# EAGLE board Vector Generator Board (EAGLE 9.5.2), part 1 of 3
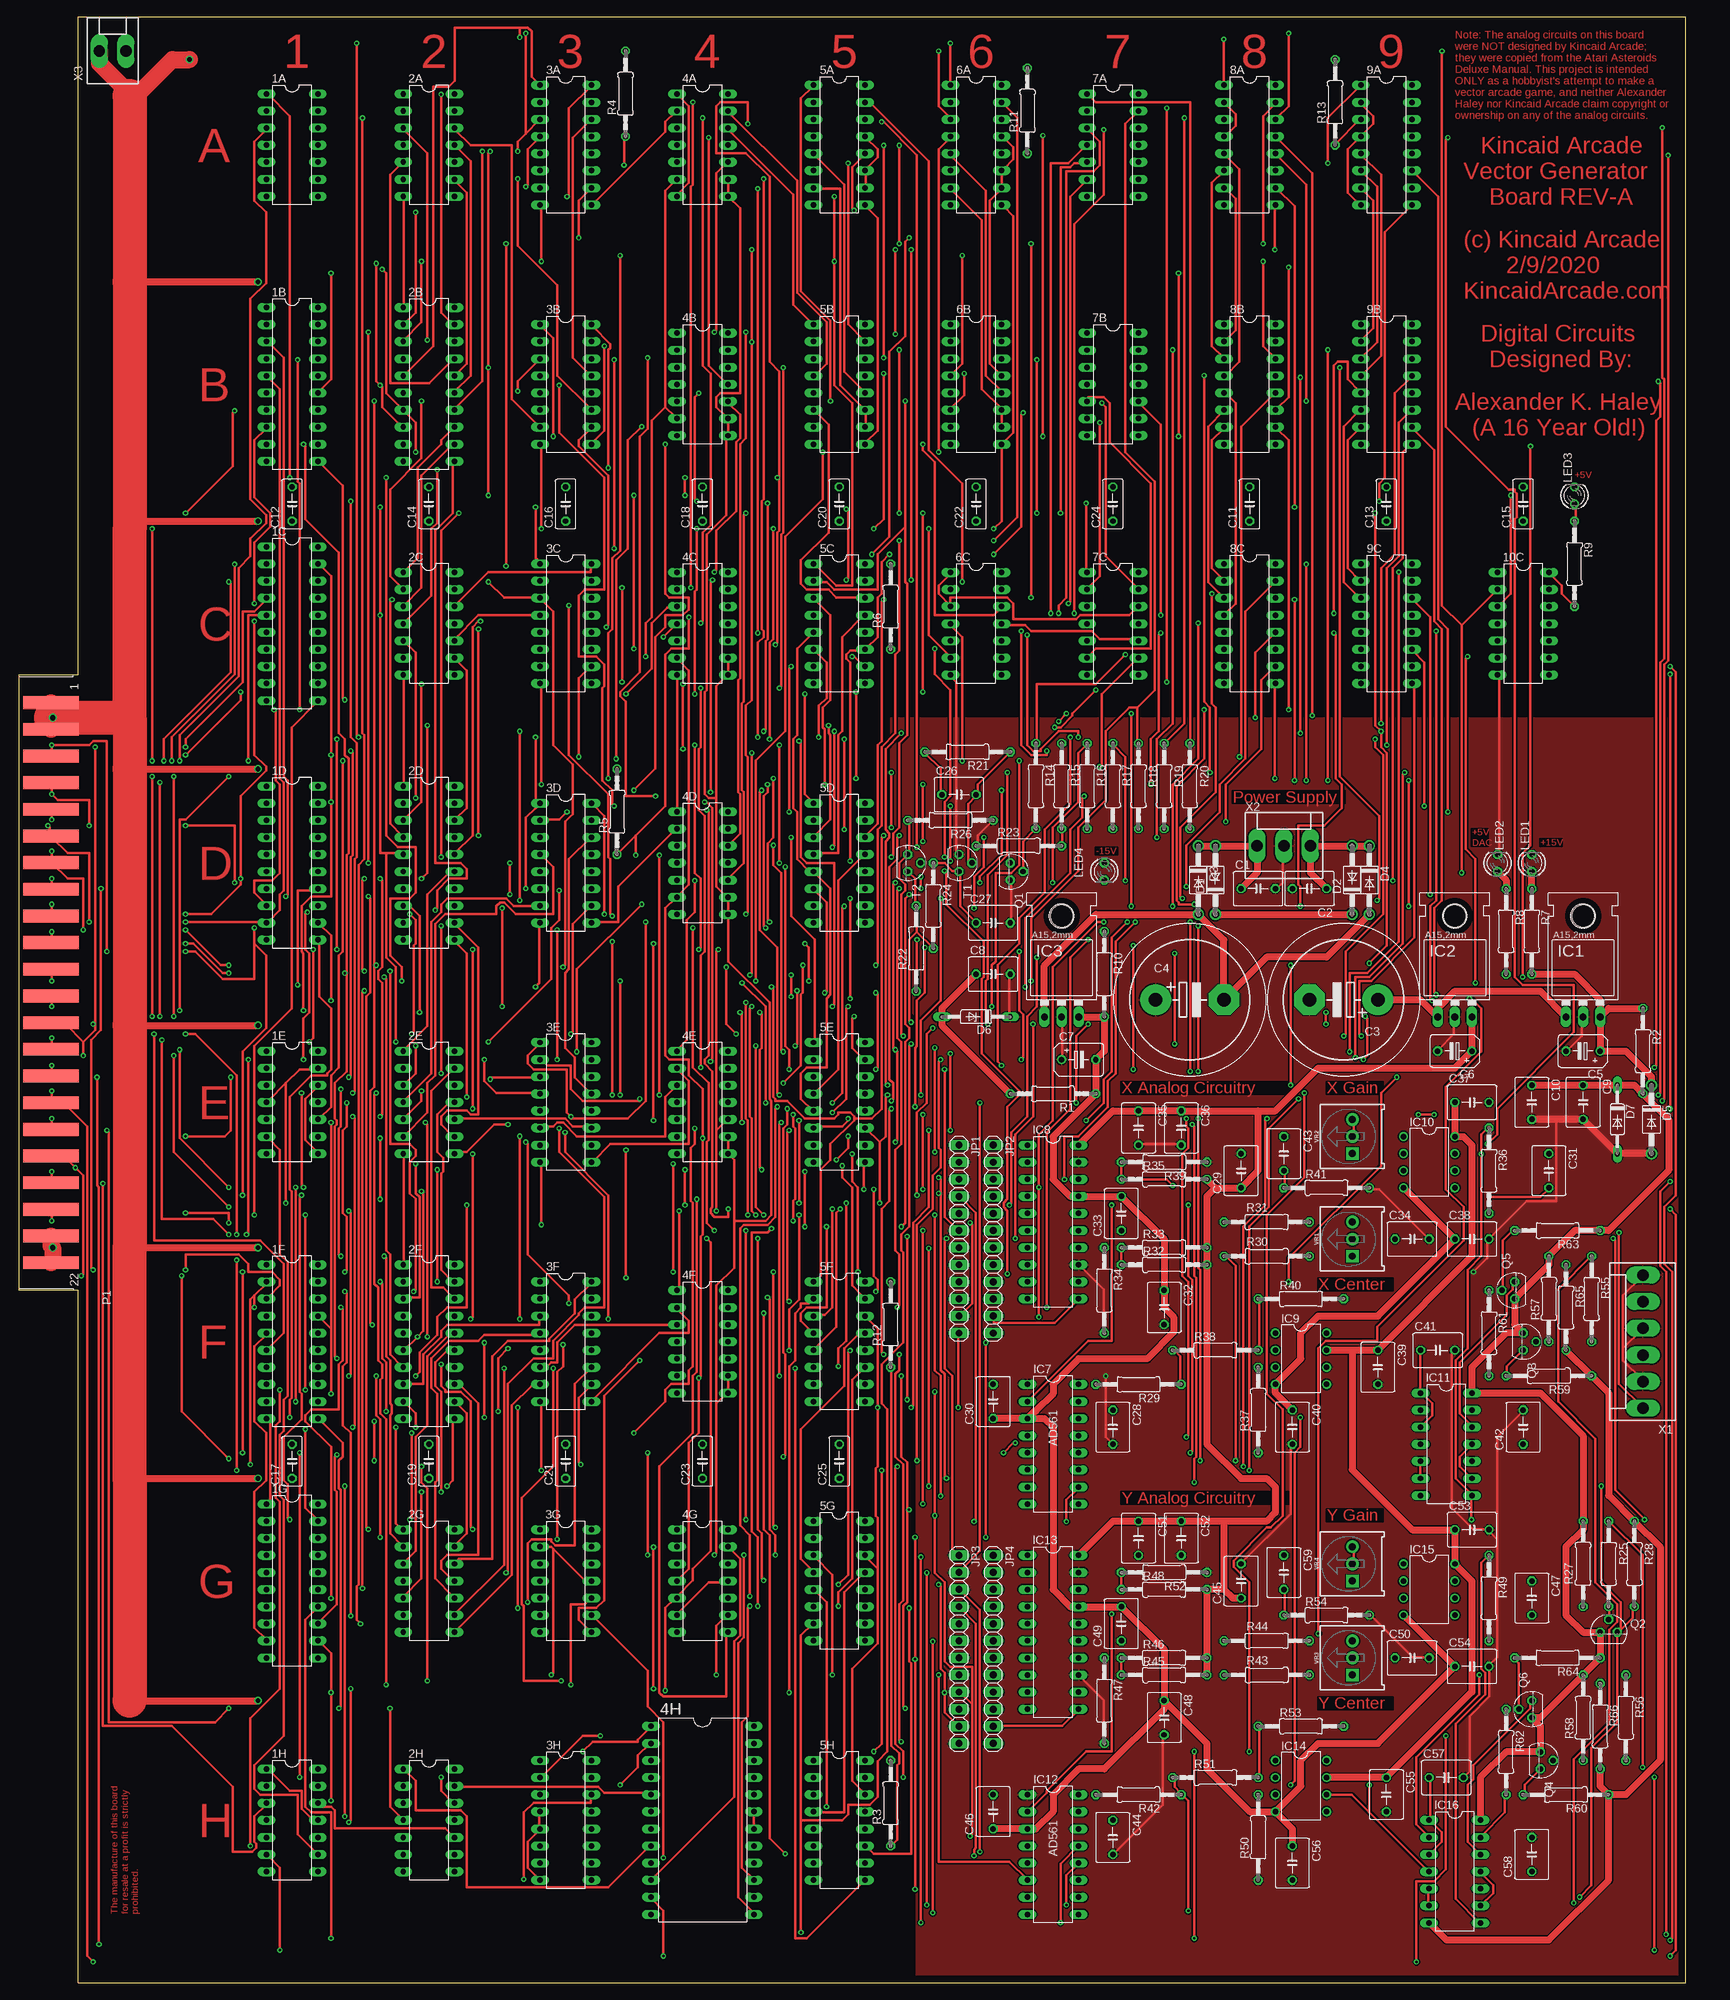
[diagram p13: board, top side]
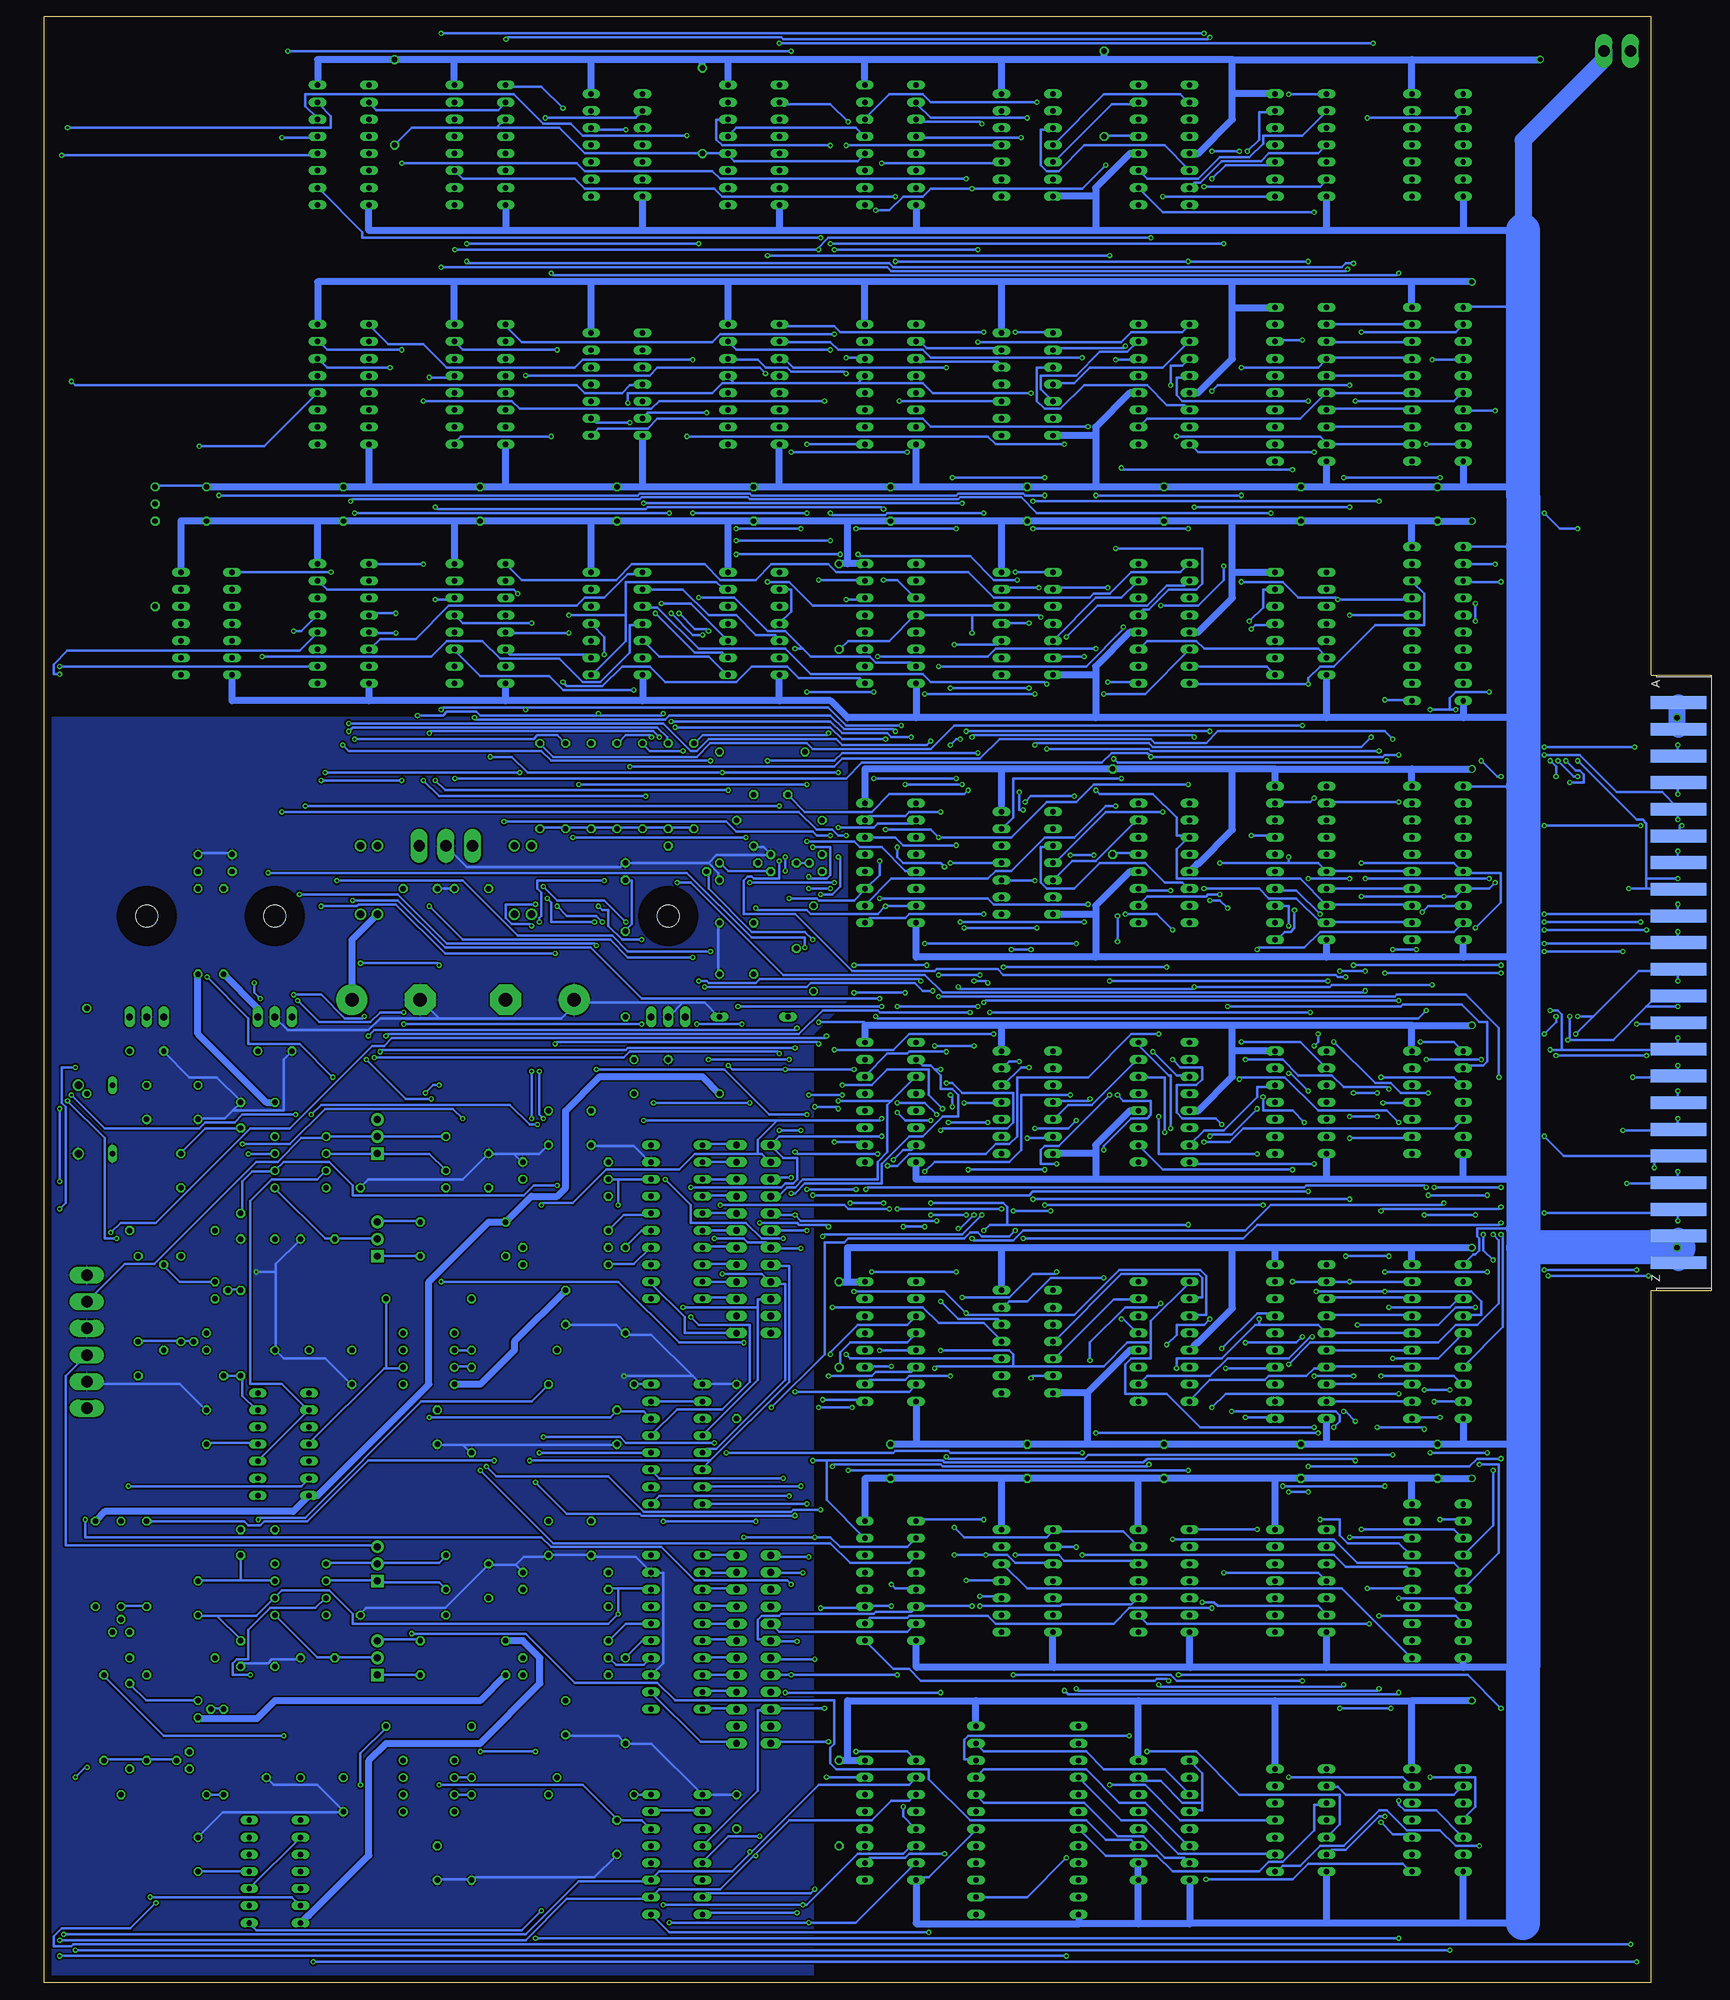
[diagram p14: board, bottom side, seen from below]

Size 247.65 x 292.1 mm. Coordinates in mm from the lower left corner, seen from the top.
Outline: 8.89,0 8.89,102.87 0,102.87 0,194.31 8.89,194.31 8.89,292.1 247.65,292.1 247.65,0 8.89,0
Copper layers (1*16): Top 0.035mm / dielectric 1.5mm / Bottom 0.035mm
Design rules "default": minimum track width 6mil, minimum drill 0.35mm, track to track 6mil, track to pad 6mil, pad to pad 6mil, via to via 6mil, smd to smd 6mil, copper to edge 40mil, drill to drill 6mil, minimum pad ring 10mil, minimum via ring 8mil, stop-mask expansion 4mil, vias tented up to drill 0mil, thermal gap 10mil
Net classes: 0 default: width 0.381 mm, clearance 0.203 mm

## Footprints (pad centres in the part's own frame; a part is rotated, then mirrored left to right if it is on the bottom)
DIL14 = drill 0.813 long: 1 -7.62,-3.81; 2 -5.08,-3.81; 3 -2.54,-3.81; 4 0,-3.81; 5 2.54,-3.81; 6 5.08,-3.81; 7 7.62,-3.81; 8 7.62,3.81; 9 5.08,3.81; 10 2.54,3.81; 11 0,3.81; 12 -2.54,3.81; 13 -5.08,3.81; 14 -7.62,3.81
DIL20 = drill 0.813 long: 1 -11.43,-3.81; 2 -8.89,-3.81; 3 -6.35,-3.81; 4 -3.81,-3.81; 5 -1.27,-3.81; 6 1.27,-3.81; 7 3.81,-3.81; 8 6.35,-3.81; 9 8.89,-3.81; 10 11.43,-3.81; 11 11.43,3.81; 12 8.89,3.81; 13 6.35,3.81; 14 3.81,3.81; 15 1.27,3.81; 16 -1.27,3.81; 17 -3.81,3.81; 18 -6.35,3.81; 19 -8.89,3.81; 20 -11.43,3.81
DIL16 = drill 0.813 long: 1 -8.89,-3.81; 2 -6.35,-3.81; 3 -3.81,-3.81; 4 -1.27,-3.81; 5 1.27,-3.81; 6 3.81,-3.81; 7 6.35,-3.81; 8 8.89,-3.81; 9 8.89,3.81; 10 6.35,3.81; 11 3.81,3.81; 12 1.27,3.81; 13 -1.27,3.81; 14 -3.81,3.81; 15 -6.35,3.81; 16 -8.89,3.81
DIL24-6 = drill 0.813 long: 1 -13.97,-7.62; 2 -11.43,-7.62; 3 -8.89,-7.62; 4 -6.35,-7.62; 5 -3.81,-7.62; 6 -1.27,-7.62; 7 1.27,-7.62; 8 3.81,-7.62; 9 6.35,-7.62; 10 8.89,-7.62; 11 11.43,-7.62; 12 13.97,-7.62; 13 13.97,7.62; 14 11.43,7.62; 15 8.89,7.62; 16 6.35,7.62; 17 3.81,7.62; 18 1.27,7.62; 19 -1.27,7.62; 20 -3.81,7.62; 21 -6.35,7.62; 22 -8.89,7.62; 23 -11.43,7.62; 24 -13.97,7.62
C050-050X075 = drill 0.813 octagon: 1 -2.54,0; 2 2.54,0
EB22,5D = drill 2.007 pad 4.597: + -5.08,0 | drill 2.007 pad 4.597 octagon: - 5.08,0
B45181B = drill 0.813: + -2.54,0 | drill 0.813 octagon: - 2.54,0
C050-030X075 = drill 0.813 octagon: 1 -2.54,0; 2 2.54,0
DO41-10 = drill 1.118: A 5.08,0; C -5.08,0
DO35Z10 = drill 0.813 long: A 5.08,0; C -5.08,0
78XXL = drill 1.016 long: GND 0,-3.81; IN -2.54,-3.81; OUT 2.54,-3.81 | hole 3.302: 0,11.176
DIL08 = drill 0.813 pad 1.27: 1 -3.81,-3.81; 2 -1.27,-3.81; 3 1.27,-3.81; 4 3.81,-3.81; 5 3.81,3.81; 6 1.27,3.81; 7 -1.27,3.81; 8 -3.81,3.81
1X12 = drill 1.016 long: 1 -13.97,0; 2 -11.43,0; 3 -8.89,0; 4 -6.35,0; 5 -3.81,0; 6 -1.27,0; 7 1.27,0; 8 3.81,0; 9 6.35,0; 10 8.89,0; 11 11.43,0; 12 13.97,0
LED3MM = drill 0.813 octagon: A -1.27,0; K 1.27,0
44PINEDGE = smd 1.905 x 8.255: 1 -41.605,4.826; 2 -37.643,4.826; 3 -33.68,4.826; 4 -29.718,4.826; 5 -25.756,4.826; 6 -21.793,4.826; 7 -17.831,4.826; 8 -13.868,4.826; 9 -9.906,4.826; 10 -5.944,4.826; 11 -1.981,4.826; 12 1.981,4.826; 13 5.944,4.826; 14 9.906,4.826; 15 13.868,4.826; 16 17.831,4.826; 17 21.793,4.826; 18 25.756,4.826; 19 29.718,4.826; 20 33.68,4.826; 21 37.643,4.826; 22 41.605,4.826 | smd 1.905 x 8.255 bottom: A -41.605,4.826; B -37.643,4.826; C -33.68,4.826; D -29.718,4.826; E -25.756,4.826; F -21.793,4.826; H -17.831,4.826; J -13.868,4.826; K -9.906,4.826; L -5.944,4.826; M -1.981,4.826; N 1.981,4.826; P 5.944,4.826; R 9.906,4.826; S 13.868,4.826; T 17.831,4.826; U 21.793,4.826; V 25.756,4.826; W 29.718,4.826; X 33.68,4.826; Y 37.643,4.826; Z 41.605,4.826
TO92 = drill 0.813 octagon: 1 1.27,0; 2 0,1.905; 3 -1.27,0
0207/12 = drill 0.813 octagon: 1 -6.35,0; 2 6.35,0
TRIMPOT-PTH-3386U = drill 1.016 pad 1.88 square: 1 -2.54,-0.015 | drill 1.016 pad 1.88: 2 0,-0.015; 3 2.54,-0.015
KK-156-6 = drill 1.7 pad 2.184 long: 1 -9.9,0; 2 -5.94,0; 3 -1.98,0; 4 1.98,0; 5 5.94,0; 6 9.9,0
KK-156-3 = drill 1.7 pad 2.184 long: 1 -3.96,0; 2 0,0; 3 3.96,0
KK-156-2 = drill 1.7 pad 2.184 long: 1 -1.98,0; 2 1.98,0

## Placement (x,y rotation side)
1A  7400N  [DIL14]  40.64,273.05 270 top
1B  74HC573N  [DIL20]  40.64,237.49 270 top
1C  74HC573N  [DIL20]  40.64,201.93 270 top
1D  74HC573N  [DIL20]  40.64,166.37 270 top
1E  74S08N  [DIL14]  40.64,130.81 270 top
1F  74HC573N  [DIL20]  40.64,95.25 270 top
1G  74HC573N  [DIL20]  40.64,59.69 270 top
1H  7432N  [DIL14]  40.64,24.13 270 top
2A  7404N  [DIL14]  60.96,273.05 270 top
2B  74HC573N  [DIL20]  60.96,237.49 270 top
2C  7404N  [DIL14]  60.96,201.93 270 top
2D  74HC573N  [DIL20]  60.96,166.37 270 top
2E  7404N  [DIL14]  60.96,130.81 270 top
2F  74HC573N  [DIL20]  60.96,95.25 270 top
2G  7404N  [DIL14]  60.96,59.69 270 top
2H  7404N  [DIL14]  60.96,24.13 270 top
3A  7483N  [DIL16]  81.28,273.05 270 top
3B  7483N  [DIL16]  81.28,237.49 270 top
3C  7483N  [DIL16]  81.28,201.93 270 top
3D  7483N  [DIL16]  81.28,166.37 270 top
3E  7483N  [DIL16]  81.28,130.81 270 top
3F  7483N  [DIL16]  81.28,95.25 270 top
3G  74S11N  [DIL14]  81.28,59.69 270 top
3H  74191N  [DIL16]  81.28,24.13 270 top
4A  7495N  [DIL14]  101.6,273.05 270 top
4B  7495N  [DIL14]  101.6,237.49 270 top
4C  7495N  [DIL14]  101.6,201.93 270 top
4D  7495N  [DIL14]  101.6,166.37 270 top
4E  7495N  [DIL14]  101.6,130.81 270 top
4F  7495N  [DIL14]  101.6,95.25 270 top
4G  7404N  [DIL14]  101.6,59.69 270 top
4H  74154N  [DIL24-6]  101.6,24.13 270 top
5A  7497N  [DIL16]  121.92,273.05 270 top
5B  7497N  [DIL16]  121.92,237.49 270 top
5C  74191N  [DIL16]  121.92,201.93 270 top
5D  74191N  [DIL16]  121.92,166.37 270 top
5E  74191N  [DIL16]  121.92,130.81 270 top
5F  74191N  [DIL16]  121.92,95.25 270 top
5G  74191N  [DIL16]  121.92,59.69 270 top
5H  74191N  [DIL16]  121.92,24.13 270 top
6A  7497N  [DIL16]  142.24,273.05 270 top
6B  7497N  [DIL16]  142.24,237.49 270 top
6C  74S11N  [DIL14]  142.24,201.93 270 top
7A  74LS27N  [DIL14]  162.56,273.05 270 top
7B  7432N  [DIL14]  162.56,237.49 270 top
7C  7404N  [DIL14]  162.56,201.93 270 top
8A  7485N  [DIL16]  182.88,273.05 270 top
8B  7485N  [DIL16]  182.88,237.49 270 top
8C  7485N  [DIL16]  182.88,201.93 270 top
9A  7485N  [DIL16]  203.2,273.05 270 top
9B  7485N  [DIL16]  203.2,237.49 270 top
9C  7485N  [DIL16]  203.2,201.93 270 top
10C  7402N  [DIL14]  223.52,201.93 270 top
C1  .1 uf  [C050-050X075]  184.15,162.56 0 top
C2  .1 uf  [C050-050X075]  191.77,162.56 180 top
C3  470 uf  [EB22,5D]  196.85,146.05 180 top
C4  470 uf  [EB22,5D]  173.99,146.05 0 top
C5  1 uf  [B45181B]  232.41,138.43 180 top
C6  1 uf  [B45181B]  213.36,138.43 180 top
C7  1 uf  [B45181B]  157.48,137.16 0 top
C8  .1 uf  [C050-050X075]  144.78,149.86 0 top
C9  .1 uf  [C050-050X075]  232.41,130.81 270 top
C10  22pf  [C050-050X075]  224.79,130.81 270 top
C11  .1uf  [C050-030X075]  182.88,219.71 90 top
C12  .1uf  [C050-030X075]  40.64,219.71 90 top
C13  .1uf  [C050-030X075]  203.2,219.71 90 top
C14  .1uf  [C050-030X075]  60.96,219.71 90 top
C15  .1uf  [C050-030X075]  223.52,219.71 90 top
C16  .1uf  [C050-030X075]  81.28,219.71 90 top
C17  .1uf  [C050-030X075]  40.64,77.47 90 top
C18  .1uf  [C050-030X075]  101.6,219.71 90 top
C19  .1uf  [C050-030X075]  60.96,77.47 90 top
C20  .1uf  [C050-030X075]  121.92,219.71 90 top
C21  .1uf  [C050-030X075]  81.28,77.47 90 top
C22  .1uf  [C050-030X075]  142.24,219.71 90 top
C23  .1uf  [C050-030X075]  101.6,77.47 90 top
C24  .1uf  [C050-030X075]  162.56,219.71 90 top
C25  .1uf  [C050-030X075]  121.92,77.47 90 top
C26  270pf  [C050-050X075]  139.7,176.53 0 top
C27  .01uf  [C050-050X075]  144.78,157.48 0 top
C28  .1uf  [C050-050X075]  162.56,82.55 270 top
C29  .1uf  [C050-050X075]  181.61,120.65 90 top
C30  .1uf  [C050-050X075]  144.78,86.36 90 top
C31  10pf  [C050-050X075]  227.33,120.65 270 top
C32  .1uf  [C050-050X075]  170.18,100.33 270 top
C33  .01uf  [C050-050X075]  163.83,114.3 90 top
C34  .1uf  [C050-050X075]  207.01,110.49 0 top
C35  .1uf  [C050-050X075]  166.37,127 270 top
C36  .1uf  [C050-050X075]  172.72,127 270 top
C37  .1uf  [C050-050X075]  215.9,130.81 0 top
C38  .1uf  [C050-050X075]  215.9,110.49 0 top
C39  .1uf  [C050-050X075]  201.93,91.44 270 top
C40  .1uf  [C050-050X075]  189.23,82.55 270 top
C41  220pf  [C050-050X075]  210.82,93.98 0 top
C42  220pf  [C050-050X075]  223.52,82.55 90 top
C43  69pf  [C050-050X075]  187.96,123.19 270 top
C44  .1uf  [C050-050X075]  162.56,21.59 270 top
C45  .1uf  [C050-050X075]  181.61,59.69 90 top
C46  .1uf  [C050-050X075]  144.78,25.4 90 top
C47  10pf  [C050-050X075]  224.79,57.15 270 top
C48  .1uf  [C050-050X075]  170.18,39.37 270 top
C49  .01uf  [C050-050X075]  163.83,53.34 90 top
C50  .1uf  [C050-050X075]  207.01,48.26 0 top
C51  .1uf  [C050-050X075]  166.37,66.04 270 top
C52  .1uf  [C050-050X075]  172.72,66.04 270 top
C53  .1uf  [C050-050X075]  215.9,67.31 0 top
C54  .1uf  [C050-050X075]  215.9,46.99 0 top
C55  .1uf  [C050-050X075]  203.2,27.94 270 top
C56  .1uf  [C050-050X075]  189.23,17.78 270 top
C57  220pf  [C050-050X075]  212.09,30.48 0 top
C58  220pf  [C050-050X075]  224.79,19.05 90 top
C59  69pf  [C050-050X075]  187.96,60.96 270 top
D1  1N4004  [DO41-10]  177.8,163.83 90 top
D2  1N4004  [DO41-10]  198.12,163.83 90 top
D3  1N4004  [DO41-10]  175.26,163.83 270 top
D4  1N4004  [DO41-10]  200.66,163.83 270 top
D5  NTE109  [DO41-10]  242.57,128.27 270 top
D6  NTE5016  [DO35Z10]  142.24,143.51 180 top
D7  1n756a  [DO35Z10]  237.49,128.27 270 top
IC1  7815  [78XXL]  232.41,147.32 0 top
IC2  7805  [78XXL]  213.36,147.32 0 top
IC3  7915  [78XXL]  154.94,147.32 0 top
IC7  AD561  [DIL16]  153.67,80.01 270 top
IC8  DAC312  [DIL20]  153.67,113.03 270 top
IC9  TL081P  [DIL08]  190.5,92.71 270 top
IC10  TL082P  [DIL08]  209.55,121.92 270 top
IC11  4016N  [DIL14]  212.09,80.01 270 top
IC12  AD561  [DIL16]  153.67,19.05 270 top
IC13  DAC312  [DIL20]  153.67,52.07 270 top
IC14  TL081P  [DIL08]  190.5,29.21 270 top
IC15  TL082P  [DIL08]  209.55,58.42 270 top
IC16  4016N  [DIL14]  213.36,16.51 270 top
JP1  [1X12]  139.7,110.49 270 top
JP2  [1X12]  144.78,110.49 270 top
JP3  [1X12]  139.7,49.53 270 top
JP4  [1X12]  144.78,49.53 270 top
LED1  [LED3MM]  224.79,166.37 90 top
LED2  [LED3MM]  219.71,166.37 90 top
LED3  [LED3MM]  231.14,220.98 90 top
LED4  [LED3MM]  161.29,165.1 270 top
P1  44PINEDGE  [44PINEDGE]  0,148.59 270 top
Q1  2N3906  [TO92]  147.32,165.1 270 top
Q2  2N3906  [TO92]  236.22,52.07 0 top
Q3  2N3906  [TO92]  223.52,95.25 270 top
Q4  2N3906  [TO92]  226.06,33.02 270 top
Q5  2N3906  [TO92]  222.25,102.87 90 top
Q6  2N3906  [TO92]  224.79,40.64 90 top
R1  270  [0207/12]  153.67,132.08 180 top
R2  270  [0207/12]  241.3,138.43 270 top
R3  1K  [0207/12]  129.54,26.67 90 top
R4  1K  [0207/12]  90.17,280.67 90 top
R5  1K  [0207/12]  88.9,173.99 90 top
R6  1K  [0207/12]  129.54,204.47 90 top
R7  680  [0207/12]  224.79,156.21 270 top
R8  150  [0207/12]  220.98,156.21 270 top
R9  150  [0207/12]  231.14,210.82 270 top
R10  680  [0207/12]  161.29,149.86 270 top
R11  1K  [0207/12]  149.86,278.13 90 top
R12  1K  [0207/12]  129.54,97.79 90 top
R13  1K  [0207/12]  195.58,279.4 90 top
R14  1.2K  [0207/12]  151.13,177.8 270 top
R15  2.2K  [0207/12]  154.94,177.8 270 top
R16  4.7K  [0207/12]  158.75,177.8 270 top
R17  10K  [0207/12]  162.56,177.8 270 top
R18  22K  [0207/12]  166.37,177.8 270 top
R19  47K  [0207/12]  170.18,177.8 270 top
R20  82K  [0207/12]  173.99,177.8 270 top
R21  1K  [0207/12]  140.97,182.88 180 top
R22  12K  [0207/12]  133.35,153.67 90 top
R23  150K  [0207/12]  148.59,168.91 0 top
R24  68  [0207/12]  135.89,160.02 270 top
R25  18K  [0207/12]  236.22,62.23 270 top
R26  27  [0207/12]  138.43,172.72 180 top
R27  2.2K  [0207/12]  232.41,62.23 90 top
R28  3.3K  [0207/12]  240.03,62.23 270 top
R29  2.2K  [0207/12]  166.37,88.9 180 top
R30  56K  [0207/12]  185.42,107.95 180 top
R31  56K  [0207/12]  185.42,113.03 0 top
R32  10k  [0207/12]  170.18,106.68 0 top
R33  10k  [0207/12]  170.18,109.22 0 top
R34  4.7K  [0207/12]  161.29,102.87 270 top
R35  10K  [0207/12]  170.18,119.38 0 top
R36  8.2K  [0207/12]  218.44,120.65 270 top
R37  4.7K  [0207/12]  184.15,85.09 90 top
R38  10K  [0207/12]  177.8,93.98 0 top
R39  2.2K  [0207/12]  170.18,121.92 180 top
R40  10K  [0207/12]  190.5,101.6 0 top
R41  3.9K  [0207/12]  194.31,118.11 0 top
R42  2.2K  [0207/12]  166.37,27.94 180 top
R43  56K  [0207/12]  185.42,45.72 180 top
R44  56K  [0207/12]  185.42,50.8 0 top
R45  10k  [0207/12]  170.18,45.72 0 top
R46  10k  [0207/12]  170.18,48.26 0 top
R47  4.7K  [0207/12]  161.29,41.91 270 top
R48  10K  [0207/12]  170.18,58.42 0 top
R49  8.2K  [0207/12]  218.44,57.15 270 top
R50  4.7K  [0207/12]  184.15,21.59 90 top
R51  10K  [0207/12]  177.8,30.48 0 top
R52  2.2K  [0207/12]  170.18,60.96 180 top
R53  10K  [0207/12]  190.5,38.1 0 top
R54  3.9K  [0207/12]  194.31,54.61 0 top
R55  18K  [0207/12]  233.68,101.6 270 top
R56  18K  [0207/12]  238.76,39.37 270 top
R57  2.2K  [0207/12]  227.33,101.6 90 top
R58  2.2K  [0207/12]  232.41,39.37 90 top
R59  3.3K  [0207/12]  227.33,90.17 180 top
R60  3.3K  [0207/12]  229.87,27.94 180 top
R61  100K  [0207/12]  218.44,96.52 270 top
R62  100K  [0207/12]  220.98,34.29 270 top
R63  4.7K  [0207/12]  228.6,111.76 180 top
R64  4.7K  [0207/12]  228.6,48.26 180 top
R65  56K  [0207/12]  229.87,100.33 270 top
R66  56K  [0207/12]  234.95,38.1 270 top
T1  2N3904  [TO92]  139.7,166.37 270 top
T2  2N3904  [TO92]  132.08,166.37 270 top
VR1  10k  [TRIMPOT-PTH-3386U]  198.12,110.49 90 top
VR2  10k  [TRIMPOT-PTH-3386U]  198.12,125.73 90 top
VR3  10k  [TRIMPOT-PTH-3386U]  198.12,48.26 90 top
VR4  10k  [TRIMPOT-PTH-3386U]  198.12,62.23 90 top
X1  [KK-156-6]  241.3,95.25 90 top
X2  [KK-156-3]  187.96,168.91 0 top
X3  [KK-156-2]  13.97,287.02 0 top

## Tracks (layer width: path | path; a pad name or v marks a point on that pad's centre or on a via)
2.5MHZ  (via drill 0.35)
  Top 0.381: v103.67,45.73 103.67,53.04 105.13,54.5 4G.9 | v60.73,44.86 60.73,73.48 59.86,74.36 v59.86,76.69 | v31.23,77.86 24.22,84.87 v24.22,105.03 | v9.32,105.03 9.61,105.32 9.61,119.93 v8.45,121.09 6.98,122.56 4.94,122.56 P1.18 | v140.18,181.56 140.18,199.96 138.43,201.71 6C.4 | v108.93,182.73 108.93,150.01 v108.64,149.72 | v114.77,146.51 v114.77,149.72 | v31.52,134.53 31.52,126.64 30.64,125.77 v24.8,125.77
  Bottom 0.381: v103.67,45.73 80.3,45.73 79.43,44.86 v60.73,44.86 | v59.86,76.69 35.9,76.69 34.73,77.86 v31.23,77.86 | v9.32,105.03 v24.22,105.03 | 6C.4 138.43,202.01 136.68,203.76 136.68,206.97 138.43,206.97 6C.2 | v140.18,181.56 130.25,181.56 129.08,182.73 v108.93,182.73 | v114.77,149.72 v108.64,149.72 | v114.77,146.51 47,146.51 46.71,146.8 36.49,146.8 31.52,141.83 v31.52,134.53 | v24.8,125.77 21.88,122.85 8.45,122.85 | 8.45,122.85 4.94,122.85 P1.18 8.45,122.85 | 8.45,122.85 v8.45,121.09
20MHZ  (via drill 0.35)
  Top 0.381: 79.43,64.43 84.1,59.75 84.98,59.75 3G.11 | 79.43,64.43 79.13,64.72 77.67,64.72 3G.2 | 79.43,64.43 79.43,46.02 v79.13,45.73 | v31.23,40.77 29.18,38.72 13.41,38.72 13.41,126.35 v13.12,126.64 | v4.94,128.4 4.94,126.94 P1.17
  Bottom 0.381: v79.13,45.73 36.2,45.73 v31.23,40.77 | v13.12,126.64 4.94,126.64 P1.17 4.94,126.94 v4.94,128.4
25VAC_A
  Top 1.016: D3.C D1.A X2.1 184,164.95 C1.1
25VAC_B
  Top 1.016: C2.1 191.92,164.95 X2.3 D2.A D4.C
+5V_DAC
  Top 1.016: IC2.OUT C6.+ 213.36,135.89 193.04,135.89 186.69,129.54 184.15,129.54 | 184.15,129.54 184.15,120.65 C29.1 177.8,118.11 | 184.15,129.54 C36.1 C35.1 162.56,129.54 IC8.20 | R35.2 177.8,118.11 | 177.8,118.11 176.53,116.84 R33.2 R32.2 176.53,80.01 181.61,74.93 185.42,74.93 186.69,73.66 186.69,69.85 185.42,68.58 179.07,68.58 | 179.07,68.58 C52.1 C51.1 162.56,68.58 IC13.20 | 179.07,68.58 179.07,58.42 | 179.07,58.42 R48.2 R46.2 R45.2 | 179.07,58.42 180.34,57.15 C45.1
  Bottom 1.016: IC2.OUT 215.9,144.78 R8.2
+5VDC  (via drill 0.35)
  Top 0.381: v188.96,29.38 189.55,29.96 189.55,78.74 190.42,79.62 v190.42,84
  Bottom 0.381: IC12.14 157.71,22.95 158.88,24.12 162.38,24.12 C44.1 162.67,24.41 167.64,29.38 v188.96,29.38 | IC7.14 157.71,84 158.59,84.87 162.38,84.87 C28.1 162.67,84.87 163.55,84 v190.42,84
+8.2VDC  (via drill 0.35)
  Top 0.381: v180.78,77.57 180.78,106.49 179.32,107.95 R30.2
  Top 1.016: C10.1 C9.1 D7.C 240.03,133.35 R2.2 245.11,128.27 245.11,120.65 236.22,111.76 R63.1 231.14,111.76 R57.2 227.33,106.68 Q5.3 222.25,97.79 Q3.3 220.98,96.52 215.9,91.44 IC11.14 226.06,87.63 232.41,81.28 R27.2 232.41,67.31 229.87,64.77 229.87,54.61 232.41,52.07 Q2.3 R64.1 R58.2 226.06,39.37 Q6.3 226.06,38.1 Q4.3 220.98,34.29 217.17,30.48 IC16.14
  Bottom 0.381: v180.78,77.57 199.48,77.57 208.53,68.52 214.96,68.52 215.54,67.93 217.3,67.93 217.88,68.52 232.19,68.52 R27.2
  Bottom 1.016: R43.2 182.88,41.91 213.36,41.91 216.05,39.22 224.64,39.22 Q6.3
+15VDC
  Top 1.016: IC1.OUT C5.+ 238.76,138.43 242.57,134.62 D5.C | IC1.OUT 236.22,144.78 R2.1 | R7.2 231.14,149.86 234.95,146.05 IC1.OUT | C37.1 IC10.8 214.63,125.73 215.9,124.46 215.9,107.95 C39.1 198.12,93.98 | 198.12,93.98 IC9.7 | 198.12,93.98 198.12,76.2 207.01,67.31 C53.1 IC15.8 215.9,59.69 215.9,43.18 C55.1 IC14.7
  Bottom 1.016: C37.1 214.63,130.81 224.79,140.97 R7.2
+22VDC
  Top 1.016: C3.+ 208.28,146.05 IC2.IN 210.82,144.78 213.36,147.32 226.06,147.32 IC1.IN | D1.C D2.C
  Bottom 1.016: D2.C 201.93,154.94 C3.+
-8.2VDC
  Top 1.016: R1.2 137.16,142.24 D6.A 137.16,144.78 C8.1 | R65.2 R59.1 236.22,87.63 236.22,72.39 R28.1 243.84,64.77 243.84,33.02 238.76,27.94 R60.1 | R60.1 234.95,29.21 R66.2 | IC16.7 212.09,6.35 227.33,6.35 236.22,15.24 R60.1
  Bottom 1.016: IC16.7 208.43,10.01 208.3,10.01 199.39,18.92 199.39,33.02 196.85,35.56 182.88,35.56 173.99,44.45 173.99,48.26 176.53,50.8 R44.1 | R28.1 238.61,70 210.67,70 IC11.7 207.01,72.39 190.5,88.9 190.5,104.14 181.61,113.03 R31.1 175.26,116.84 171.45,116.84 170.18,118.11 170.18,129.54 165.1,134.62 149.86,134.62 R1.2
-15VDC
  Top 1.016: IC3.OUT R10.2 161.29,138.43 C7.- R1.1 153.67,125.73 153.67,119.38 156.21,116.84 IC8.17 C33.2 170.18,110.49 C32.1 170.18,100.33 171.6,98.91 171.6,96.67 167.64,92.71 157.48,92.71 153.67,88.9 153.67,87.5 151.11,84.94 150.98,84.94 IC7.3 | IC7.3 C30.1 | IC7.3 152.4,83.82 153.67,82.55 153.67,58.42 156.21,55.88 IC13.17 C49.2 170.18,49.53 C48.1 | C48.1 170.18,40.64 161.29,31.75 157.48,31.75 153.67,27.94 153.67,25.4 151.13,22.86 IC12.3 C46.1 | C48.1 176.53,35.56 176.53,31.75 182.88,25.4 IC14.4 | IC14.4 189.23,22.86 C56.1 | IC14.4 190.5,29.21 190.5,33.02 193.04,35.56 201.93,35.56 C54.1 IC15.4 | C40.1 186.69,87.63 IC9.4 190.5,92.71 190.5,96.52 193.04,99.06 201.93,99.06 C38.1 IC10.4
  Bottom 1.016: C32.1 177.8,95.25 177.8,93.98 182.88,88.9 IC9.4
/BEAMOFF
  Top 0.381: 7C.6 158.88,197.04 160.05,198.21 168.22,198.21 168.22,222.75 162.09,228.88 162.09,234.72 161.21,235.6 158.88,235.6 158.88,235.01 7B.5
/COUNT  (via drill 0.35)
  Top 0.381: v108.64,55.96 108.34,55.66 108.34,39.6 107.47,38.72 107.47,17.11 109.22,15.35 4H.15 | 6A.13 146.32,274.15 147.78,272.69 147.78,270.94 146.32,269.48 6A.11 146.03,269.19 146.03,266.85 6A.10 146.03,266.56 144.27,264.81 144.27,240.56 146.03,238.81 6B.13 | 5A.10 125.87,266.85 125.87,269.19 5A.11 125.87,269.48 127.62,271.23 127.62,272.4 125.87,274.15 5A.13 | v160.92,234.72 161.51,234.14 161.51,211.94 166.18,207.26 7C.13 | v82.06,44.27 82.06,56.25 84.1,56.25 84.98,57.12 3G.10 | v54.6,44.27 54.6,83.71 53.72,84.58 53.72,89.55 54.01,89.84 54.01,91.88 53.43,92.47 53.43,103.28 52.84,103.86 52.84,131.9 v53.14,132.19 | v49.63,132.19 49.92,132.49 49.92,166.95 50.22,167.25 50.22,184.19 49.34,185.06 v49.34,220.12 | v100.75,220.12 100.46,220.41 100.46,235.6 v101.04,236.18
  Bottom 0.381: v108.64,55.96 96.66,55.96 96.37,56.25 86.14,56.25 85.27,57.12 3G.10 | 6A.13 146.03,274.45 144.86,275.62 127.04,275.62 125.87,274.45 5A.13 | 126.75,237.64 125.87,238.52 5B.13 | 145.15,237.64 126.75,237.64 | 145.15,237.64 146.03,238.52 6B.13 | v160.92,234.72 160.92,236.18 148.36,236.18 146.9,237.64 145.15,237.64 | v82.06,44.27 81.76,43.98 54.89,43.98 v54.6,44.27 | v49.63,132.19 v53.14,132.19 | v100.75,220.12 v49.34,220.12 | v101.04,236.18 115.65,236.18 117.11,237.64 126.75,237.64
/FRAMECOMPLETE  (via drill 0.35)
  Top 0.381: 4G.6 97.83,54.79 102.5,59.46 105.13,59.46 4G.11 | 39.7,133.66 41.75,135.7 44.37,135.7 1E.13 | 39.7,133.66 37.07,131.03 1E.4 | v110.68,59.75 110.39,60.05 110.39,66.76 109.8,67.35 v109.8,110.58 | 39.7,133.66 v39.7,115.84
  Bottom 0.381: v110.68,59.75 105.42,59.75 4G.11 | v109.8,110.58 109.51,110.29 103.67,110.29 102.21,111.75 69.2,111.75 65.41,115.55 39.99,115.55 v39.7,115.84
/HALTROTATE  (via drill 0.35)
  Top 0.381: v205.03,209.6 205.03,154.69 200.35,150.01 197.73,150.01 v197.73,138.33 | v136.09,123.43 v136.09,138.91 | v123.83,123.14 123.83,119.05 124.7,118.17 v124.7,105.61 | v112.14,105.61 112.14,67.93 v112.43,67.64
  Bottom 0.381: 3G.13 85.27,65.01 87.31,67.06 97.54,67.06 4G.1 97.83,67.06 98.7,66.18 110.97,66.18 v112.43,67.64 | v205.03,209.6 219.63,209.6 10C.1 | v197.73,138.33 197.43,138.62 161.21,138.62 160.92,138.91 v136.09,138.91 | v136.09,123.43 135.8,123.14 v123.83,123.14 | v112.14,105.61 v124.7,105.61
/INHIBITX  (via drill 0.35)
  Top 0.381: v169.69,203.18 169.69,231.51 166.47,234.72 7B.10
  Bottom 0.381: 161.21,203.18 161.21,208.14 147.78,208.14 146.9,207.26 146.32,207.26 6C.13 | 161.21,203.18 161.21,199.38 166.18,194.41 7C.8 | 161.21,203.18 v169.69,203.18
/INHIBITY  (via drill 0.35)
  Top 0.381: v160.63,231.8 160.63,209.02 158.88,207.26 7C.2
  Bottom 0.381: 6C.5 138.43,199.67 139.01,200.25 141.94,200.25 144.86,203.18 148.95,203.18 152.74,206.97 158.59,206.97 7C.2 | v160.63,231.8 165.59,231.8 166.18,232.38 7B.9
/LDCOUNTERS  (via drill 0.35)
  Top 0.381: v123.53,166.66 123.53,196.16 122.95,196.75 122.95,197.33 123.53,197.92 125.58,197.92 5C.11 125.87,198.21 127.62,199.96 127.62,205.8 128.21,206.39 128.21,211.06 v129.38,212.23 | v149.24,233.26 148.95,232.97 148.95,216.32 v144.86,212.23 | v132.3,55.66 132.3,47.78 132.59,47.48 132.59,19.15 127.04,19.15 125.87,20.32 5H.11 | v121.78,55.96 121.78,58 123.83,60.05 123.83,89.55 125.58,91.3 5F.11 | 127.91,124.89 125.87,126.94 5E.11 | v127.91,115.84 127.91,124.89 | v122.95,115.84 122.95,95.39 121.78,94.22 v121.78,91.59 | v136.97,161.11 136.97,145.92 134.05,143 v134.05,131.9 | v129.08,131.9 128.79,131.61 128.79,125.77 127.91,124.89
  Bottom 0.381: v123.53,166.66 123.53,164.62 125.58,162.57 5D.11 125.87,162.28 127.33,160.82 132.59,160.82 132.88,161.11 v136.97,161.11 | v149.24,233.26 158,233.26 158.59,232.68 7B.6 | v129.38,212.23 v144.86,212.23 | v132.3,55.66 125.87,55.66 5G.11 125.58,55.96 v121.78,55.96 | v122.95,115.84 v127.91,115.84 | v121.78,91.59 125.58,91.59 5F.11 | v129.08,131.9 v134.05,131.9
/LDROT  (via drill 0.35)
  Top 0.381: v107.76,63.55 107.76,51.28 106.88,50.41 106.88,12.73 109.22,10.39 4H.13 | v40.28,223.62 40.28,277.37 37.07,280.58 1A.1 | v54.6,223.62 54.6,170.46 56.35,168.71 58.98,168.71 58.98,161.99 58.1,161.11 55.18,161.11 55.18,152.64 56.93,150.89 v56.93,148.84 | v89.36,131.9 v89.36,148.84 | v97.24,105.61 v97.24,121.68 | v111.27,101.82 111.56,101.52 111.56,67.35 112.43,66.47 v112.43,63.55
  Bottom 0.381: 4G.3 97.83,62.38 103.38,62.38 104.55,63.55 v107.76,63.55 v112.43,63.55 | v54.6,223.62 v40.28,223.62 | v89.36,148.84 v56.93,148.84 | v89.36,131.9 96.95,124.31 99,124.31 99.58,123.72 99.58,121.68 v97.24,121.68 | v97.24,105.61 97.54,105.32 100.75,105.32 104.25,101.82 v111.27,101.82
/LDX2
  Bottom 0.381: 2H.9 64.82,19.15 79.13,19.15 84.1,24.12 87.61,24.12 93.74,30.25 4H.4
/LDXY1  (via drill 0.35)
  Top 0.381: v83.81,34.34 85.27,35.8 91.99,35.8 91.99,36.09 93.74,37.85 4H.1
  Bottom 0.381: v83.81,34.34 76.5,34.34 70.08,27.92 55.18,27.92 55.18,23.53 56.93,21.78 2H.5
/LDY2
  Bottom 0.381: 4H.7 93.74,22.66 89.94,18.86 82.35,18.86 80.01,16.52 67.16,16.52 65.7,17.98 63.65,17.98 58.98,22.66 58.98,26.45 57.23,26.45 2H.3
/LDZ
  Top 0.381: 4H.10 94.03,15.35 106.3,27.62 106.3,50.7 107.17,51.58 107.17,62.97 105.42,64.72 4G.13
/ROTATE  (via drill 0.35)
  Top 0.381: v95.78,18.57 95.78,38.72 93.45,41.06 93.45,46.32 85.27,54.5 3G.9 | v51.09,277.08 51.09,185.65 51.38,185.36 51.38,166.95 50.51,166.08 50.51,59.17 50.22,58.88 50.22,53.91 v50.8,53.33
  Bottom 0.381: v95.78,18.57 101.62,12.73 109.22,12.73 4H.14 | v51.09,277.08 37.95,277.08 37.07,277.95 1A.2 | v50.8,53.33 83.81,53.33 3G.9
/SUBTRACT  (via drill 0.35)
  Top 0.381: v95.78,3.96 95.78,10.68 94.03,12.43 4H.11 | v245.34,3.96 246.22,4.84 246.22,114.08 v245.34,114.96 | v243,135.99 243.29,136.28 243.29,232.09 243.88,232.68 243.88,237.64 v243.59,237.94
  Bottom 0.381: v245.34,3.96 v95.78,3.96 | v245.34,114.96 244.46,115.84 244.46,130.15 245.05,130.73 245.05,135.99 v243,135.99 | v243.59,237.94 243,237.35 168.52,237.35 167.35,236.18 161.8,236.18 160.63,237.35 158.88,237.35 7B.4
/TTLINVX  (via drill 0.35)
  Top 0.381: v231.03,11.85 231.03,33.17 236.28,38.43 236.28,52.45 237.45,53.62 237.45,56.25 234.24,59.46 234.24,80.78 228.69,86.34 228.69,102.98 233.66,107.95 R55.1 | v11.95,5.72 11.95,118.17 11.66,118.47 v11.66,134.53 | v4.94,136.28 4.94,134.82 P1.15
  Bottom 0.381: v231.03,11.85 234.82,8.05 245.05,8.05 246.22,6.88 246.22,5.42 243.59,5.42 243.29,5.72 v11.95,5.72 | v11.66,134.53 4.94,134.53 P1.15 4.94,134.82 v4.94,136.28
/TTLINVY  (via drill 0.35)
  Top 0.381: v212.04,36.68 212.04,16.81 210.29,15.06 207.66,15.06 v207.66,3.09 | v11.07,3.09 10.2,3.96 10.2,127.23 6.69,130.73 4.94,130.73 P1.16 4.94,131.03 v4.94,132.49
  Bottom 0.381: v212.04,36.68 229.86,36.68 238.62,45.44 R56.1 | v11.07,3.09 v207.66,3.09 | v4.94,132.49 4.94,131.03 P1.16
/VECTORCOMPLETE  (via drill 0.35)
  Top 0.381: v193.05,51.87 193.05,94.22 194.22,95.39 201.82,95.39 201.82,97.43 214.67,110.29 214.67,115.25 212.04,117.88 212.04,133.07 217.3,138.33 217.3,144.75 215.84,146.22 v215.54,146.22 | v216.42,148.55 216.42,166.95 214.96,168.42 214.96,196.75 v215.25,197.04
  Bottom 0.381: v193.05,51.87 176.11,51.87 168.81,44.56 156.54,44.56 153.91,41.94 130.25,41.94 130.25,35.51 130.84,34.92 130.84,32.59 129.96,31.71 116.23,31.71 116.23,30.25 110.1,24.12 92.86,24.12 89.94,21.2 86.14,21.2 85.27,20.32 3H.11 | v215.54,146.22 216.42,147.09 v216.42,148.55 | v215.25,197.04 190.13,197.04 187.8,199.38 182.54,199.38 179.91,196.75 171.15,196.75 167.64,193.24 165.01,193.24 160.63,197.62 160.63,201.71 158.88,201.71 7C.4
/VRAMPC1  (via drill 0.35)
  Top 0.381: v89.36,29.38 91.99,32 91.99,33.76 93.74,35.51 4H.2
  Bottom 0.381: v89.36,29.38 84.1,29.38 78.84,24.12 64.82,24.12 2H.11
/VRAMPC2
  Top 0.381: 4H.5 93.74,28.21 87.02,28.21 86.14,29.08 64.82,29.08 2H.13
/VRAMPC3
  Top 0.381: 4H.8 93.74,20.32 87.61,14.19 66.57,14.19 66.57,24.7 65.7,25.58 58.98,25.58 58.98,29.96 57.23,31.71 2H.1
/XCUR1
  Bottom 0.381: 3A.11 84.98,269.19 83.81,268.02 76.21,268.02 73,271.23 68.62,271.23 66.57,273.28 66.57,274.45 60.73,274.45 57.23,277.95 2A.2
/XCUR2
  Bottom 0.381: 3A.7 77.38,266.85 76.8,267.44 75.92,267.44 72.71,270.65 66.87,270.65 65.7,271.82 58.39,271.82 57.23,272.99 2A.4
/XCUR3  (via drill 0.35)
  Top 0.381: v75.34,266.85 75.63,267.14 75.63,272.4 77.38,274.15 3A.4
  Bottom 0.381: v75.34,266.85 58.1,266.85 57.23,267.73 2A.6
/XCUR4  (via drill 0.35)
  Top 0.381: v81.47,265.39 81.76,265.68 81.76,278.54 84.98,281.75 3A.16
  Bottom 0.381: v81.47,265.39 64.82,265.39 2A.8
/XCUR5  (via drill 0.35)
  Top 0.381: v74.17,268.02 74.17,258.09 80.01,252.25 80.01,238.81 84.98,233.84 3B.11
  Bottom 0.381: v74.17,268.02 72.12,270.07 65.11,270.07 64.82,270.36 2A.10
/XCUR6
  Top 0.381: 2A.12 64.82,275.32 67.16,272.99 73.29,272.99 73.29,235.31 77.38,231.22 3B.7
/XCUR7  (via drill 0.35)
  Top 0.381: v59.86,235.01 59.86,226.54 55.18,221.87 55.18,209.02 56.93,207.26 2C.2
  Bottom 0.381: v59.86,235.01 78.55,235.01 79.43,235.89 79.43,238.52 77.67,238.52 3B.4
/XCUR8  (via drill 0.35)
  Top 0.381: 2C.4 61.32,206.1 61.32,216.03 62.19,216.9 v62.19,224.79 | v87.61,225.08 87.61,242.61 87.9,242.9 87.9,243.48 85.27,246.11 3B.16
  Bottom 0.381: v62.19,224.79 87.31,224.79 v87.61,225.08
/XCUR9
  Bottom 0.381: 2C.6 57.23,197.04 58.39,198.21 75.34,198.21 76.5,199.38 83.81,199.38 84.98,198.21 3C.11
/XCUR10
  Bottom 0.381: 3C.7 65.99,195.58 64.82,194.41 2C.8
/XCUR11
  Top 0.381: 2C.10 64.82,199.67 68.33,203.18 77.38,203.18 3C.4
/XCUR12
  Top 0.381: 2C.12 64.82,204.63 69.79,209.6 84.98,209.6 84.98,210.77 3C.16
/YCUR1  (via drill 0.35)
  Top 0.381: v69.79,139.79 79.13,149.14 79.13,156.73 80.3,157.9 v80.3,162.28
  Bottom 0.381: v69.79,139.79 61.02,139.79 57.23,135.99 2E.2 | v80.3,162.28 84.98,162.28 3D.11
/YCUR2
  Top 0.381: 2E.4 57.23,131.03 61.32,135.12 61.32,157.61 62.78,159.07 62.78,160.24 63.65,161.11 72.42,161.11 73.58,159.94 77.38,159.94 3D.7
/YCUR3
  Top 0.381: 2E.6 57.23,125.77 60.73,129.27 60.73,133.66 61.9,134.82 61.9,157.31 63.36,158.78 70.95,158.78 70.95,159.94 71.54,160.53 72.12,160.53 73.88,158.78 79.43,158.78 79.43,165.79 77.67,167.54 3D.4
/YCUR4  (via drill 0.35)
  Top 0.381: v72.71,127.52 70.66,127.52 66.57,123.43 64.82,123.43 2E.8 | v80.01,156.44 v80.01,137.16 | v87.02,158.78 87.02,173.38 85.27,175.13 3D.16
  Bottom 0.381: v72.71,127.52 73.58,128.4 78.55,128.4 79.43,129.27 79.43,133.36 76.5,133.36 75.63,134.24 75.63,135.99 78.84,135.99 v80.01,137.16 | v80.01,156.44 82.35,158.78 v87.02,158.78
/YCUR5
  Top 0.381: 3E.11 84.98,127.23 82.35,127.23 81.18,128.4 64.82,128.4 2E.10
/YCUR6
  Bottom 0.381: 3E.7 77.38,124.6 75.34,126.64 72.42,126.64 67.45,131.61 67.45,133.07 64.82,133.07 2E.12
/YCUR7  (via drill 0.35)
  Top 0.381: v54.31,107.95 54.6,107.66 54.6,93.05 55.18,92.47 55.18,86.04 55.47,85.75 55.47,84.58 55.18,84.29 55.18,66.76 56.93,65.01 2G.2 | v47.88,107.95 47.59,108.24 47.59,126.94 47.88,127.23 v47.88,132.78 | v69.2,137.16 69.2,133.95 70.95,132.19 77.38,132.19 3E.4
  Bottom 0.381: v47.88,107.95 v54.31,107.95 | v47.88,132.78 48.17,133.07 54.6,133.07 56.35,134.82 61.32,134.82 63.65,137.16 v69.2,137.16
/YCUR8  (via drill 0.35)
  Top 0.381: v72.42,60.92 72.71,61.21 72.71,88.96 76.5,92.76 79.43,92.76 79.43,95.39 83.22,99.19 83.22,99.48 84.1,100.36 87.02,100.36 87.02,116.71 80.3,123.43 v80.3,126.94
  Bottom 0.381: v72.42,60.92 58.39,60.92 57.23,59.75 2G.4 | v80.3,126.94 80.3,134.82 80.59,134.82 85.27,139.5 3E.16
/YCUR9  (via drill 0.35)
  Top 0.381: v75.63,56.54 75.63,65.3 76.21,65.89 79.13,65.89 79.13,65.6 79.72,65.01 82.64,65.01 82.64,88.96 84.98,91.3 3F.11
  Bottom 0.381: v75.63,56.54 73.88,56.54 73.29,55.96 58.39,55.96 57.23,54.79 2G.6
/YCUR10
  Top 0.381: 2G.8 64.82,52.16 73.29,60.63 73.29,85.75 76.21,88.67 77.38,88.67 3F.7
/YCUR11
  Top 0.381: 2G.10 64.53,57.42 61.9,60.05 61.9,74.36 62.19,74.65 62.19,87.5 61.32,88.38 61.32,92.76 63.94,95.39 68.33,95.39 69.2,96.27 77.38,96.27 3F.4
/YCUR12
  Top 0.381: 2G.12 64.82,62.38 65.41,62.97 70.37,62.97 70.37,93.05 72.71,95.39 78.84,95.39 78.84,95.68 82.64,99.48 82.64,101.52 84.98,103.86 3F.16
A  (via drill 0.35)
  Top 0.381: R52.2 163.84,60.92 163.84,58.59 R48.1 | v162.38,54.79 162.38,34.34 158.59,34.34 152.74,28.5 152.74,28.21 150.11,25.58 IC12.2
  Bottom 0.381: 221.97,54.5 218.47,50.99 R49.2 | 221.97,54.5 224.6,54.5 C47.2 | 221.97,54.5 216.13,54.5 213.5,57.12 IC15.6 213.21,57.42 212.33,58.29 205.32,58.29 201.82,54.79 201.82,53.33 163.84,53.33 v162.38,54.79 162.38,58.59 | IC12.2 150.11,25.58 157.42,25.58 IC12.15 | 162.38,58.59 163.55,58.59 R48.1 | 162.38,58.59 157.71,58.59 IC13.18
B  (via drill 0.35)
  Top 0.381: C31.2 227.23,117.88 226.06,116.71 218.47,116.71 218.47,114.38 R36.2 | R39.2 163.84,121.68 163.84,119.63 R35.1 163.84,119.34 170.56,119.34 v171.44,118.47 | v162.38,115.55 162.38,95.39 158.88,95.39 150.11,86.63 IC7.2
  Bottom 0.381: R36.2 218.17,114.38 218.17,119.05 216.71,120.51 213.5,120.51 IC10.6 212.04,121.97 205.32,121.97 201.82,118.47 201.82,117 176.4,117 174.94,118.47 v171.44,118.47 | IC7.2 150.11,86.34 157.42,86.34 IC7.15 | 162.38,119.34 163.55,119.34 R35.1 | 162.38,119.34 157.71,119.34 IC8.18 | 162.38,119.34 v162.38,115.55
BRMSACTIVE  (via drill 0.35)
  Top 0.381: v48.17,181.56 48.17,153.22 47.59,152.64 47.59,135.99 46.42,134.82 46.42,130.15 44.67,128.4 1E.10 | v88.77,181.85 88.77,211.35 90.53,213.11 90.53,229.17 v92.57,231.22
  Bottom 0.381: v48.17,181.56 48.46,181.27 88.19,181.27 v88.77,181.85 | v92.57,231.22 115.94,231.22 117.11,232.38 156.54,232.38 158,230.92 165.3,230.92 166.18,230.05 7B.8
COUNT
  Top 0.381: 138.43,204.63 136.68,206.39 136.68,207.56 138.43,209.31 6C.1 | 138.43,204.63 138.43,205.8 146.9,205.8 147.78,204.93 147.78,202.59 157.12,202.59 157.71,203.18 165.01,203.18 166.18,204.34 7C.12 | 138.43,204.63 6C.3
DACX1  (via drill 0.35)
  Top 0.381: v122.95,208.43 123.24,208.72 123.24,218.66 v122.95,218.95 | v189.55,219.24 189.55,263.93 186.92,266.56 8A.10 | v139.6,85.46 139.6,96.27 JP1.12 | v103.38,111.75 102.21,112.92 102.21,124.89 102.5,125.18 102.5,133.66 100.17,135.99 v100.17,156.73 | v110.97,156.73 110.68,157.02 110.68,176.3 111.27,176.89 v111.27,178.05 | v119.74,178.05 119.74,186.23 119.44,186.53 119.44,189.45 120.61,190.61 120.61,203.18 118.28,205.51 5C.3
  Bottom 0.381: v122.95,208.43 120.9,208.43 118.28,205.8 5C.3 | v122.95,218.95 123.24,219.24 158,219.24 158.29,218.95 189.25,218.95 v189.55,219.24 | v139.6,85.46 131.71,93.34 131.71,110 128.79,110 128.21,110.58 110.97,110.58 110.1,111.45 108.93,111.45 108.34,110.87 104.25,110.87 v103.38,111.75 | v110.97,156.73 v100.17,156.73 | v119.74,178.05 v111.27,178.05
DACX2  (via drill 0.35)
  Top 0.381: 131.71,216.32 127.62,212.23 127.62,206.97 121.2,206.97 120.03,208.14 118.28,208.14 5C.2 | v131.71,235.01 131.71,216.32 | v191.3,235.01 191.3,267.14 186.92,271.53 8A.12 | v141.35,112.92 141.64,112.62 141.64,100.94 139.89,99.19 JP1.11 | v131.13,112.33 131.71,112.92 131.71,139.79 132.3,140.37 132.3,141.83 131.71,142.42 131.71,161.11 v132.3,161.7 | v129.67,167.25 129.96,167.54 129.96,170.75 130.84,171.63 130.84,184.19 132,185.36 132,207.85 131.71,208.14 131.71,216.32
  Bottom 0.381: v131.71,235.01 156.25,235.01 157.42,233.84 176.99,233.84 178.16,235.01 v191.3,235.01 | v141.35,112.92 135.8,112.92 135.51,112.62 131.42,112.62 v131.13,112.33 | v132.3,161.7 130.54,161.7 129.38,162.87 129.38,167.25 v129.67,167.25
DACX3  (via drill 0.35)
  Top 0.381: v118.86,185.06 118.86,189.74 120.03,190.91 120.03,196.16 118.28,197.92 5C.6 | v155.66,188.57 v154.5,187.4 | v192.18,188.28 192.18,268.9 186.92,274.15 8A.13 | v152.74,100.36 152.74,126.35 156.25,129.86 156.25,152.35 v158.88,154.98 | v165.3,188.57 v165.3,159.94
  Bottom 0.381: 141.64,100.36 141.64,101.52 139.89,101.52 JP1.10 | 141.64,100.36 141.64,89.55 149.82,81.37 IC7.4 | v118.86,185.06 121.78,185.06 122.37,185.65 129.08,185.65 130.84,187.4 v154.5,187.4 | v155.66,188.57 155.96,188.28 165.3,188.28 | 165.3,188.28 182.83,188.28 183.41,188.86 187.8,188.86 188.38,188.28 v192.18,188.28 | v152.74,100.36 141.64,100.36 | v158.88,154.98 161.8,154.98 163.84,157.02 163.84,159.36 164.72,159.36 v165.3,159.94 | 165.3,188.28 v165.3,188.57
DACX4  (via drill 0.35)
  Top 0.381: v150.41,258.38 v150.41,205.8 | v184.87,258.38 184.87,277.37 186.63,279.12 8A.15 | v146.9,105.32 146.9,114.67 146.32,115.25 146.32,115.84 146.9,116.42 146.9,130.15 148.65,131.9 148.65,132.49 143.1,138.04 143.1,149.14 143.4,149.43 143.4,154.69 137.85,160.24 137.85,164.91 v137.55,165.2 | v137.55,167.25 137.55,175.43 138.43,176.3 138.43,192.07 136.09,194.41 v136.09,198.21
  Bottom 0.381: IC7.5 149.82,78.74 149.24,79.32 147.78,79.32 137.55,89.55 137.55,103.86 139.6,103.86 JP1.9 139.89,104.15 141.06,105.32 v146.9,105.32 | 134.92,198.21 137.55,200.84 140.18,200.84 145.15,205.8 v150.41,205.8 | 134.92,198.21 133.76,197.04 124.99,197.04 124.12,196.16 118.86,196.16 118.28,195.58 5C.7 | v184.87,258.38 v150.41,258.38 | v137.55,167.25 v137.55,165.2 | 134.92,198.21 v136.09,198.21
DACX5  (via drill 0.35)
  Top 0.381: v120.32,186.82 120.32,185.65 120.61,185.36 120.61,172.8 118.28,170.46 5D.3 | v188.67,189.15 188.67,229.17 186.92,230.92 8B.10 | v175.53,77.57 175.53,105.91 175.24,106.2 v175.24,128.4 | v175.24,157.02 v175.24,135.41 | v174.65,160.24 172.31,160.24 172.31,160.53 172.02,160.82 172.02,177.76 176.11,181.85 v176.11,189.15
  Bottom 0.381: 148.65,77.57 136.97,89.26 136.97,106.49 139.6,106.49 JP1.8 | 148.65,77.57 149.82,76.4 IC7.6 | v120.32,186.82 128.5,186.82 131.13,189.45 176.11,189.45 | 176.11,189.45 188.38,189.45 v188.67,189.15 | v175.53,77.57 148.65,77.57 | v175.24,135.41 v175.24,128.4 | v175.24,157.02 175.53,157.31 178.16,157.31 179.03,158.19 179.03,160.24 v174.65,160.24 | 176.11,189.45 v176.11,189.15
DACX6  (via drill 0.35)
  Top 0.381: v135.22,109.12 v135.22,73.77 | v129.67,179.81 v129.67,171.63 | v181.37,182.14 181.66,182.44 181.66,231.22 186.63,236.18 8B.12 | v148.07,110.58 148.07,126.06 150.7,128.69 v150.7,142.42 | v143.98,142.42 143.69,142.71 143.69,148.84 143.98,149.14 143.98,164.62 146.9,167.54 v146.9,179.81
  Bottom 0.381: v135.22,73.77 149.82,73.77 IC7.7 | v135.22,109.12 139.6,109.12 JP1.7 140.47,110 143.1,110 143.69,110.58 v148.07,110.58 | v129.67,171.63 124.41,171.63 123.83,172.21 118.57,172.21 118.28,172.5 5D.2 | v129.67,179.81 v146.9,179.81 175.82,179.81 178.16,182.14 v181.37,182.14 | v143.98,142.42 v150.7,142.42
DACX7  (via drill 0.35)
  Top 0.381: v119.74,147.09 120.03,147.38 120.03,160.53 118.28,162.28 5D.6 | v127.33,147.09 127.62,146.8 127.62,135.99 v127.33,135.7 | v137.55,135.7 137.55,113.79 139.6,111.75 JP1.6 | v134.34,111.75 v134.34,71.14 | v190.42,185.65 v190.42,238.52 | v156.25,185.06 156.25,175.13 152.45,171.34 152.45,161.99 148.65,158.19 148.65,154.39 145.44,151.18 145.44,136.87 v146.03,136.28
  Bottom 0.381: v127.33,147.09 v119.74,147.09 | v127.33,135.7 v137.55,135.7 145.44,135.7 v146.03,136.28 | v134.34,71.14 149.82,71.14 IC7.8 | v134.34,111.75 139.6,111.75 JP1.6 | v190.42,238.52 186.92,238.52 8B.13 | v190.42,185.65 190.13,185.94 157.12,185.94 v156.25,185.06
DACX8  (via drill 0.35)
  Top 0.381: v136.97,72.31 136.97,90.13 136.09,91.01 v136.09,114.08 | v122.66,159.94 122.37,159.65 122.37,132.19 v120.9,130.73 | v115.06,128.98 115.06,127.23 115.35,126.94 115.35,116.42 115.06,116.13 v115.06,113.21 | v171.44,242.61 171.44,187.11 169.1,184.77 v169.1,170.17 | v143.4,170.17 143.4,165.79 141.94,164.32 v141.94,159.65
  Bottom 0.381: v136.97,72.31 156.25,72.31 157.42,71.14 IC7.9 | JP1.5 139.6,114.08 v136.09,114.08 135.22,113.21 v115.06,113.21 | v120.9,130.73 116.81,130.73 v115.06,128.98 | 5D.7 118.28,159.94 v122.66,159.94 123.83,158.78 133.76,158.78 134.34,159.36 141.64,159.36 v141.94,159.65 | 8B.15 185.46,242.61 v171.44,242.61 | v143.4,170.17 v169.1,170.17
DACX9  (via drill 0.35)
  Top 0.381: v155.66,68.52 155.66,71.73 157.42,73.48 IC7.10 | v141.94,68.52 142.23,68.81 142.23,114.38 139.89,116.71 JP1.4 | v179.32,172.5 179.32,178.05 184.58,183.31 184.58,193.53 186.63,195.58 8C.10 | v130.84,170.46 130.54,170.17 130.54,166.95 129.38,165.79 129.38,134.24 129.96,133.66 129.96,131.32 v129.67,131.03
  Bottom 0.381: v141.94,68.52 v155.66,68.52 | 121.78,131.03 122.37,130.44 122.37,123.43 123.83,121.97 123.83,119.34 134.92,119.34 136.09,118.17 137.26,118.17 138.43,117 139.6,117 JP1.4 | 121.78,131.03 118.28,134.53 5E.3 | v179.32,172.5 146.32,172.5 144.86,171.04 133.46,171.04 132.88,170.46 v130.84,170.46 | 121.78,131.03 v129.67,131.03
DACX10  (via drill 0.35)
  Top 0.381: v137.85,74.94 137.55,75.23 137.55,90.42 136.97,91.01 136.97,117.3 | 136.97,117.3 136.97,119.34 v136.68,119.63 | 136.97,117.3 v136.68,117.3 | v183.71,187.99 183.71,197.62 186.63,200.55 8C.12 | v121.2,185.94 121.2,169 v120.9,168.71 | v113.89,165.79 113.89,139.2 114.48,138.62 v114.48,135.7
  Bottom 0.381: v137.85,74.94 156.25,74.94 157.42,76.11 IC7.11 | v136.68,119.63 139.6,119.63 JP1.3 | 115.35,135.7 114.48,134.82 114.48,132.78 112.73,132.78 111.85,131.9 111.85,128.69 114.19,128.69 117.11,125.77 119.15,125.77 123.24,121.68 123.24,118.76 134.63,118.76 136.09,117.3 v136.68,117.3 | 115.35,135.7 115.94,136.28 117.11,136.28 117.98,137.16 5E.2 | v183.71,187.99 183.41,187.69 155.37,187.69 154.79,188.28 130.84,188.28 128.79,186.23 121.49,186.23 v121.2,185.94 | v120.9,168.71 120.9,167.25 120.03,166.37 114.48,166.37 v113.89,165.79 | 115.35,135.7 v114.48,135.7
DACX11  (via drill 0.35)
  Top 0.381: v174.07,78.74 174.36,79.03 174.36,104.44 173.77,105.03 v173.77,115.55 | v123.24,128.4 123.24,128.11 122.37,127.23 118.28,127.23 5E.6 | v175.24,202.01 175.24,181.85 171.44,178.05 v171.44,159.94 | v164.72,157.61 162.38,155.27 162.38,135.41 161.21,134.24 161.21,130.73 v158.59,128.11
  Bottom 0.381: v174.07,78.74 IC7.12 | v173.77,115.55 173.48,115.84 169.1,115.84 164.13,120.8 153.33,120.8 150.99,123.14 141.64,123.14 | 141.64,123.14 141.06,123.14 139.89,121.97 JP1.2 | v123.24,128.4 123.53,128.11 138.72,128.11 | 138.72,128.11 141.64,125.18 141.64,123.14 | v175.24,202.01 185.46,202.01 186.63,203.18 8C.13 | v171.44,159.94 169.98,158.48 165.59,158.48 v164.72,157.61 | 138.72,128.11 v158.59,128.11
DACX12  (via drill 0.35)
  Top 0.381: v151.57,98.9 v151.57,118.17 151.57,126.06 153.62,128.11 153.62,150.89 160.34,157.61 v161.21,157.61 | v121.49,122.26 123.24,124.02 v123.24,125.77 | v173.48,162.87 173.48,169 178.45,173.97 178.45,178.05 182.25,181.85 182.25,203.76 186.63,208.14 8C.15
  Bottom 0.381: v151.57,98.9 150.41,97.73 142.81,97.73 142.81,89.26 146.9,85.17 153.62,85.17 157.42,81.37 IC7.13 | v151.57,118.17 138.14,118.17 137.55,118.76 136.38,118.76 135.8,119.34 135.8,122.56 137.85,122.56 139.6,124.31 JP1.1 139.6,124.6 138.43,125.77 v123.24,125.77 | v121.49,122.26 120.03,123.72 118.86,123.72 118.28,124.31 5E.7 | v173.48,162.87 171.44,160.82 164.43,160.82 v161.21,157.61
DACY1  (via drill 0.35)
  Top 0.381: v130.84,93.34 130.84,91.01 130.25,90.42 130.25,78.16 131.42,76.99 131.42,56.83 130.84,56.25 130.84,36.09 v131.13,35.8 | v132.3,259.26 131.71,258.67 131.71,244.65 129.38,242.32 129.38,214.86 v126.75,212.23 | v103.09,208.43 102.79,208.14 v102.79,176.89 | v102.21,174.26 102.5,173.97 102.5,137.74 101.92,137.16 101.92,136.58 103.09,135.41 103.09,115.25 102.79,114.96 102.79,114.38 103.38,113.79 105.42,113.79 v105.42,114.96 | v120.9,114.96 120.9,100.36 119.74,99.19 118.28,99.19 5F.3
  Bottom 0.381: 5F.3 119.44,97.73 126.75,97.73 130.84,93.64 v130.84,93.34 | v131.13,35.8 139.6,35.8 JP3.12 | v132.3,259.26 200.35,259.26 200.35,260.13 206.78,266.56 9A.10 | v126.75,212.23 126.45,211.94 110.1,211.94 106.59,208.43 v103.09,208.43 | v102.79,176.89 102.79,174.26 v102.21,174.26 | v120.9,114.96 v105.42,114.96
DACY2  (via drill 0.35)
  Top 0.381: v114.48,43.1 114.48,91.59 115.35,92.47 115.35,99.48 116.23,100.36 116.23,100.94 117.4,100.94 117.98,101.52 5F.2 | JP3.11 139.6,38.14 137.55,40.18 v137.55,43.1 137.55,46.02 136.97,46.61 136.97,58.88 v136.68,59.17 | v245.05,271.53 245.05,196.46 244.46,195.87 244.46,131.32 v244.17,131.03 | v236.87,110.58 237.16,110.29 237.16,73.19 v241.54,68.81
  Bottom 0.381: v137.55,43.1 v114.48,43.1 | v245.05,271.53 207.07,271.53 9A.12 | v244.17,131.03 238.62,125.48 238.62,110.58 v236.87,110.58 | v241.54,68.81 241.54,66.18 173.77,66.18 172.31,64.72 155.96,64.72 150.99,59.75 137.26,59.75 v136.68,59.17
DACY3  (via drill 0.35)
  Top 0.381: v131.13,90.13 131.13,78.16 132,77.28 132,70.27 | 132,70.27 132,56.54 131.42,55.96 131.42,41.06 v131.71,40.77 | v212.33,274.15 212.04,273.86 212.04,231.22 221.39,221.87 222.26,221.87 222.26,221.58 222.56,221.28 222.56,217.78 222.26,217.49 222.26,149.43 223.43,148.26 231.03,148.26 231.03,141.25 219.63,129.86 219.63,126.06 v218.17,124.6 | v185.46,128.4 185.17,128.11 185.17,115.55 181.95,112.33 v181.95,76.69 | 132,70.27 v132.3,70.27
  Bottom 0.381: IC12.4 149.82,20.32 141.64,28.5 141.64,40.48 139.89,40.48 JP3.10 139.6,40.77 v131.71,40.77 | v131.13,90.13 124.7,90.13 124.12,90.72 118.86,90.72 118.28,91.3 5F.6 | v212.33,274.15 207.07,274.15 9A.13 | v218.17,124.6 211.16,124.6 205.91,129.86 186.92,129.86 v185.46,128.4 | v181.95,76.69 180.49,75.23 163.84,75.23 158.59,69.98 136.68,69.98 136.38,70.27 v132.3,70.27
DACY4  (via drill 0.35)
  Top 0.381: v141.35,21.78 141.64,22.07 141.64,41.35 | 141.64,41.35 139.89,43.1 JP3.9 | v136.09,87.8 v136.09,69.39 136.09,60.92 137.55,59.46 137.55,47.78 138.43,46.9 141.64,46.9 141.64,41.35 | v244.17,275.62 244.17,238.52 244.46,238.23 244.46,196.75 243.88,196.16 243.88,132.19 v243.59,131.9 | v207.95,128.98 v210.29,128.98 | v174.36,127.52 174.65,127.23 174.65,105.03 174.94,104.74 174.94,78.16 174.65,77.86 v174.65,74.36
  Bottom 0.381: v141.35,21.78 146.03,21.78 149.82,17.98 IC12.5 | v136.09,87.8 119.15,87.8 118.28,88.67 5F.7 | v244.17,275.62 205.03,275.62 205.03,277.37 206.78,279.12 9A.15 | v243.59,131.9 238.62,126.94 224.6,126.94 223.72,127.81 219.34,127.81 218.17,128.98 v210.29,128.98 | v207.95,128.98 206.49,130.44 178.45,130.44 175.53,127.52 v174.36,127.52 | v174.65,74.36 169.98,69.69 159.17,69.69 158.88,69.39 v136.09,69.39
DACY5  (via drill 0.35)
  Top 0.381: v120.9,45.73 120.9,60.63 118.28,63.26 5G.3 | v136.68,45.73 136.68,17.98 147.19,17.98 149.82,15.35 IC12.6 | v210.58,146.8 210.29,147.09 210.29,159.65 211.46,160.82 211.46,201.13 210.29,202.3 210.29,227.71 207.07,230.92 9B.10 | v200.06,143.59 200.35,143.29 200.35,137.74 v199.77,137.16 | v190.13,131.32 185.75,126.94 185.75,115.25 182.83,112.33 v182.83,76.11
  Bottom 0.381: v120.9,45.73 v136.68,45.73 139.6,45.73 JP3.8 | v210.58,146.8 206.49,146.8 202.98,143.29 200.35,143.29 v200.06,143.59 | v199.77,137.16 193.93,131.32 v190.13,131.32 | v182.83,76.11 172.02,65.3 130.84,65.3 127.91,62.38 119.15,62.38 118.28,63.26 5G.3
DACY6  (via drill 0.35)
  Top 0.381: v133.17,13.89 v133.17,48.07 v133.17,66.18 | v224.6,228.29 224.6,169 223.43,167.83 v223.43,149.43 | v204.74,134.53 202.4,132.19 202.4,121.39 188.67,107.66 v188.67,104.15 | v143.69,66.18 v143.69,95.1
  Bottom 0.381: v133.17,13.89 133.76,13.31 149.24,13.31 149.82,12.73 IC12.7 | v133.17,48.07 139.6,48.07 JP3.7 | 5G.2 118.28,65.89 119.44,64.72 129.38,64.72 130.84,66.18 v133.17,66.18 v143.69,66.18 | v224.6,228.29 214.96,228.29 207.07,236.18 9B.12 | v223.43,149.43 217.3,143.29 217.3,139.5 209.7,139.5 v204.74,134.53 | v188.67,104.15 162.38,104.15 153.33,95.1 v143.69,95.1
DACY7  (via drill 0.35)
  Top 0.381: v135.8,50.7 v135.8,10.39 | v202.4,187.11 202.4,210.19 204.44,212.23 204.44,236.18 206.78,238.52 9B.13 | v115.94,184.48 116.23,184.19 116.23,167.25 117.11,166.37 121.2,166.37 121.2,145.34 v120.9,145.05 | v108.93,145.05 108.64,144.75 108.64,128.69 108.93,128.4 108.93,114.67 v109.51,114.08 | v111.85,112.04 111.27,111.45 108.93,111.45 108.93,67.06 109.8,66.18 v109.8,55.96
  Bottom 0.381: v135.8,10.39 149.82,10.39 IC12.8 | v135.8,50.7 139.6,50.7 JP3.6 139.89,50.99 141.64,50.99 141.64,53.91 141.06,54.5 138.43,54.5 138.14,54.79 124.41,54.79 124.12,55.08 118.86,55.08 118.28,55.66 5G.6 117.98,55.96 v109.8,55.96 | v202.4,187.11 155.66,187.11 151.57,183.02 150.7,183.02 148.95,184.77 129.96,184.77 129.08,183.9 116.52,183.9 v115.94,184.48 | v108.93,145.05 v120.9,145.05 | v109.51,114.08 111.56,112.04 v111.85,112.04
DACY8  (via drill 0.35)
  Top 0.381: 116.23,24.12 116.23,51.58 117.98,53.33 5G.7 | 116.23,24.12 v116.23,7.47 | v194.51,178.64 v194.51,242.61 | v206.49,159.94 v206.49,178.64 | v171.73,139.5 v171.73,152.93 | v132.59,139.5 132.3,139.2 132.3,112.33 131.13,111.16 131.13,108.83 131.42,108.53 131.42,95.1 128.21,91.88 128.21,86.04 129.08,85.17 129.08,34.34 127.62,32.88 127.62,27.62 126.45,26.45 123.24,26.45 123.24,24.99 122.37,24.12 116.23,24.12
  Bottom 0.381: 5G.7 118.28,53.33 119.44,52.16 138.43,52.16 139.6,53.33 JP3.5 | IC12.9 154.79,7.47 v116.23,7.47 | v194.51,242.61 205.61,242.61 206.78,243.78 9B.15 | v206.49,178.64 v194.51,178.64 | v206.49,159.94 201.23,159.94 200.94,160.24 195.39,160.24 188.09,152.93 v171.73,152.93 | v171.73,139.5 171.44,139.79 132.88,139.79 v132.59,139.5
DACY9  (via drill 0.35)
  Top 0.381: v245.34,195.58 246.22,194.7 246.22,117 244.46,115.25 244.46,106.78 245.63,105.61 245.63,6.59 v245.34,6.3 | v141.94,18.86 141.94,19.74 142.23,20.03 142.23,53.33 139.89,55.66 JP3.4
  Bottom 0.381: 142.23,18.86 147.19,13.89 156.25,13.89 157.42,12.73 IC12.10 157.71,12.43 169.98,12.43 176.11,6.3 v245.34,6.3 | 142.23,18.86 136.97,24.12 124.7,24.12 121.78,27.04 119.15,27.04 118.28,27.92 5H.3 | v245.34,195.58 9C.10 | 142.23,18.86 v141.94,18.86
DACY10  (via drill 0.35)
  Top 0.381: v245.34,129.86 v245.34,194.41 | v245.34,119.05 243.88,117.59 243.88,106.49 244.75,105.61 v244.75,7.18 | v142.81,19.44 142.81,55.37 139.89,58.29 JP3.3
  Bottom 0.381: 142.52,19.44 132.59,29.38 119.15,29.38 118.28,30.25 5H.2 | 142.52,19.44 145.44,16.52 156.25,16.52 157.42,15.35 IC12.11 157.71,15.06 168.22,15.06 176.11,7.18 v244.75,7.18 | v245.34,194.41 246.22,194.41 246.22,195.87 244.17,197.92 209.7,197.92 207.07,200.55 9C.12 | v245.34,119.05 v245.34,129.86 | 142.52,19.44 v142.81,19.44
DACY11  (via drill 0.35)
  Top 0.381: v155.66,11.56 155.66,15.94 157.42,17.69 IC12.12 | v210.58,200.84 210.58,160.82 209.7,159.94 209.7,146.22 v210,145.92 | v194.22,142.42 v194.22,144.17 | v158.88,142.42 157.12,140.67 v157.12,130.73 | v142.81,130.73 142.81,64.14 139.89,61.21 JP3.2 | v134.92,60.92 v134.92,11.56
  Bottom 0.381: v155.66,11.56 v134.92,11.56 134.34,11.56 126.75,19.15 120.03,19.15 118.86,20.32 5H.6 | v210.58,200.84 209.41,200.84 207.07,203.18 9C.13 | v210,145.92 206.78,142.71 199.19,142.71 197.73,144.17 v194.22,144.17 | v158.88,142.42 v194.22,142.42 | v142.81,130.73 v157.12,130.73 | v134.92,60.92 139.6,60.92 JP3.2
DACY12  (via drill 0.35)
  Top 0.381: v154.79,8.93 154.79,17.69 157.42,20.32 IC12.13 | v177.28,206.39 177.28,190.03 177.86,189.45 177.86,176.89 172.61,171.63 172.61,161.4 v172.9,161.11 | v165.89,157.61 162.97,154.69 162.97,135.12 161.8,133.95 161.8,130.15 157.42,125.77 155.37,125.77 v155.37,119.34 | v137.85,110.58 137.55,110.29 137.55,91.3 138.72,90.13 138.72,64.43 139.6,63.55 JP3.1 | v134.05,63.26 v134.05,8.93
  Bottom 0.381: v154.79,8.93 v134.05,8.93 127.04,8.93 118.28,17.69 5H.7 | v177.28,206.39 177.86,206.97 205.61,206.97 206.78,208.14 9C.15 | v172.9,161.11 172.31,160.53 172.31,157.61 v165.89,157.61 | v155.37,119.34 151.57,115.55 151.57,112.92 143.4,112.92 141.06,110.58 v137.85,110.58 | v134.05,63.26 139.6,63.26 JP3.1
DX1
  Top 0.381: 3A.9 85.27,264.22 96.08,275.03 96.08,276.49 97.54,277.95 4A.2
DX2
